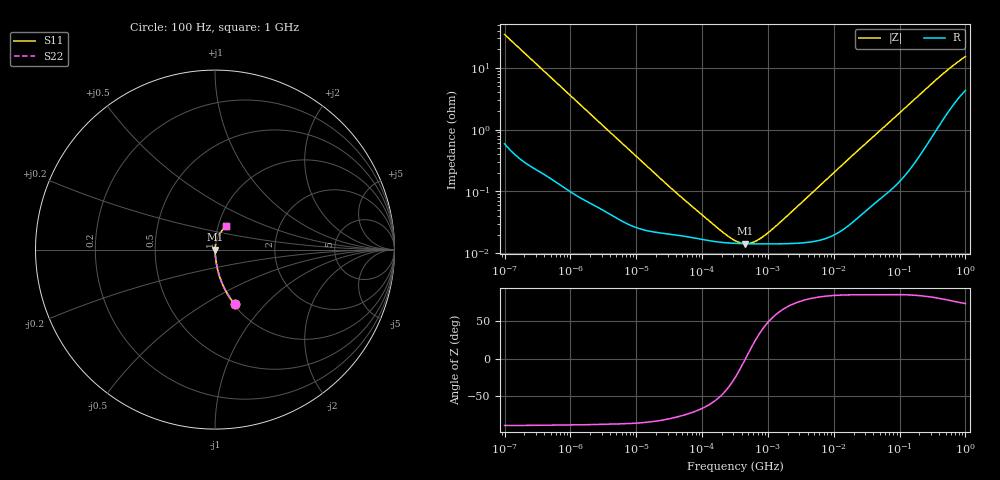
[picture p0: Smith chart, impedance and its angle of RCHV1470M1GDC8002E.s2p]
! RCHV1470M1GDC8002E  S-PARAMETER MODEL  (AEC-Q200 qualified)
! Model Generated by ELNA Corporation (http://www.ty-top.com)
! Version 1.0
! ELNA Control No. 240229
! Copyright (c) 2024 ELNA CO.,LTD. All Rights Reserved.
! Products Name : CONDUCTIVE POLYMER HYBRID ALUMINUM ELECTROLYTIC CAPACITORS
! Characteristics :
!  Capacitance  :  47uF  ,  Rated voltage  :  35V
!  Operating Temp. Range  :  -55 to +105 degC  ,  Endurance  :  10000hr at 105 degC
!  Dimension D  :  6.3mm  ,  Dimension L  :  5.8mm
! Frequency Range : 100Hz - 1GHz
! External Node Assignments :
!  1  o---| |---o  2
# MHz S RI R 50
!Freq[MHz].  S11 Real  S11 Imag  S21 Real  S21 Imag  S12 Real  S12 Imag  S22 Real  S22 Imag
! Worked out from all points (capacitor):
!   401 points, 100 Hz to 1 GHz, reference 50 ohm
!   read as one part in series: C = 46 uF near 108 Hz
!   lowest |Z| = 14.3 mohm at 454.5 kHz (marker M1)
!   series resonance near 456.4 kHz, so ESL is about 2.6 nH
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0.0001  0.1111 -0.3058  0.8889 0.3058  0.8889 0.3058  0.1111 -0.3058
0.000113  0.0899 -0.2778  0.9101 0.2778  0.9101 0.2778  0.0899 -0.2778
0.000169  0.0434 -0.1957  0.9566 0.1957  0.9566 0.1957  0.0434 -0.1957
0.000335  0.0127 -0.1025  0.9873 0.1025  0.9873 0.1025  0.0127 -0.1025
0.000638  0.00436 -0.0547  0.9956 0.0547  0.9956 0.0547  0.00436 -0.0547
0.001488  0.00133 -0.0239  0.9987 0.0239  0.9987 0.0239  0.00133 -0.0239
0.022131  0.000217 -0.00168  0.9998 0.00168  0.9998 0.00168  0.000217 -0.00168
0.049545  0.000192 -0.000765  0.9998 0.000765  0.9998 0.000765  0.000192 -0.000765
0.165959  0.000153 -0.000215  0.9998 0.000215  0.9998 0.000215  0.000153 -0.000215
0.238506  0.000147 -0.000127  0.9999 0.000127  0.9999 0.000127  0.000147 -0.000127
0.316228  0.000145 -6.88e-05  0.9999 6.88e-05  0.9999 6.88e-05  0.000145 -6.88e-05
0.386812  0.000143 -3.05e-05  0.9999 3.05e-05  0.9999 3.05e-05  0.000143 -3.05e-05
0.454465  0.000143 -7.81e-07  0.9999 7.81e-07  0.9999 7.81e-07  0.000143 -7.81e-07
0.627336  0.000142 5.96e-05  0.9999 -5.96e-05  0.9999 -5.96e-05  0.000142 5.96e-05
0.901571  0.000141 0.000135  0.9999 -0.000135  0.9999 -0.000135  0.000141 0.000135
1.522299  0.000142 0.00028  0.9999 -0.00028  0.9999 -0.00028  0.000142 0.00028
4.704354  0.000154 0.000941  0.9998 -0.000941  0.9998 -0.000941  0.000154 0.000941
69.9842  0.00117 0.0131  0.9988 -0.0131  0.9988 -0.0131  0.00117 0.0131
176.8072  0.0041 0.0321  0.9959 -0.0321  0.9959 -0.0321  0.0041 0.0321
395.8221  0.0159 0.0674  0.9841 -0.0674  0.9841 -0.0674  0.0159 0.0674
668.3439  0.0359 0.1017  0.9641 -0.1017  0.9641 -0.1017  0.0359 0.1017
1000  0.0597 0.1319  0.9403 -0.1319  0.9403 -0.1319  0.0597 0.1319
